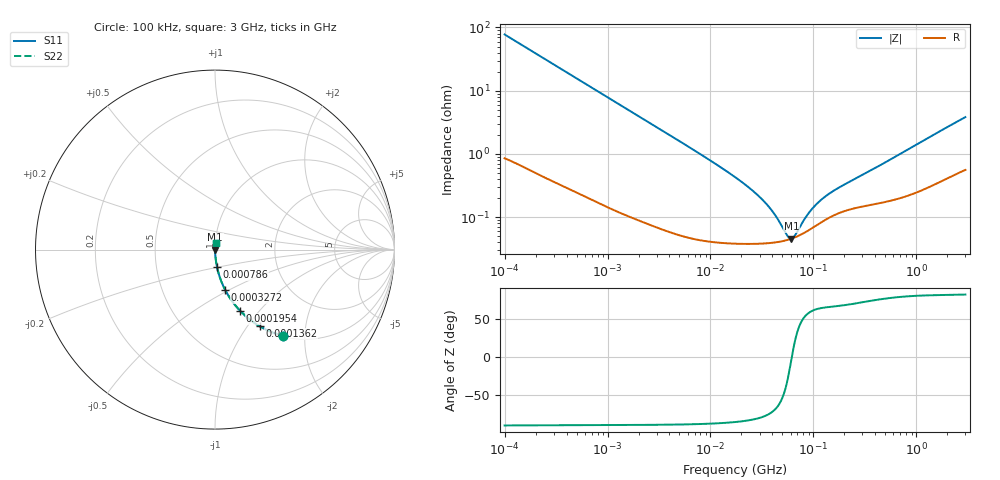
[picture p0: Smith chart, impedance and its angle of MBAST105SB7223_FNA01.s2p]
! MBAST105SB7223_FNA01  S-PARAMETER MODEL  ( Standard Model )
! Model Generated by TAIYO YUDEN Corporation (http://www.ty-top.com)
! Version 1.0
! TAIYO YUDEN Control No. 220601
! Copyright(c) 2015 TAIYO YUDEN CO.,LTD. All Rights Reserved.
! Product Description (link to TY-COMPAS)
! https://ds.yuden.co.jp/TYCOMPAS/or/detail?pn=MBAST105SB7223KFNA01&u=M
! Products Name : Multilayer Ceramic Capacitors
! Characteristics :
!  Capacitance : 0.022 [uF] , Rated Voltage : 25 [V] , TCC : X7R
!  Case Size : 1.0 x 0.5 / 0.039 x 0.02 [mm/inch] , Thickness : 0.5 / 0.02 [mm/inch]
!  (Conditions: Temperature = 25 [degC] , DC Bias Voltage = 0 [V])
! External Node Assignments :
!  1  o---| |---o  2
! GND o---------o GND
! Frequency Range : 100kHz  -  3GHz  [ 401 STEP ]
# MHZ S RI R 50
! Freq[MHz].  S11 Real  S11 Imag  S21 Real  S21 Imag  S12 Real  S12 Imag  S22 Real  S22 Imag
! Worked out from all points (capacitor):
!   401 points, 100 kHz to 3 GHz, reference 50 ohm
!   read as one part in series: C = 20.5 nF near 105.3 kHz
!   lowest |Z| = 45.8 mohm at 61.24 MHz (marker M1)
!   series resonance near 61.76 MHz, so ESL is about 320 pH
!   S11 on the Smith chart (normalised r, x): 100 kHz: 1.02, -1.55; 136.2 kHz: 1.01, -1.14; 195.4 kHz: 1.01, -0.80; 327.2 kHz: 1.01, -0.48; 786 kHz: 1.00, -0.20; 3 GHz: 1.01, +0.08
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0.1  0.3766 -0.479  0.6234 0.479  0.6234 0.479  0.3766 -0.479
0.136243  0.248 -0.4259  0.752 0.4259  0.752 0.4259  0.248 -0.4259
0.19544  0.1403 -0.341  0.8597 0.341  0.8597 0.341  0.1403 -0.341
0.327242  0.0569 -0.2247  0.9431 0.2247  0.9431 0.2247  0.0569 -0.2247
0.562235  0.0213 -0.1366  0.9787 0.1366  0.9787 0.1366  0.0213 -0.1366
0.786003  0.0116 -0.099  0.9884 0.099  0.9884 0.099  0.0116 -0.099
3.161081  0.0013 -0.0252  0.9987 0.0252  0.9987 0.0252  0.0013 -0.0252
9.331111  0.000485 -0.00843  0.9995 0.00843  0.9995 0.00843  0.000485 -0.00843
17.7727  0.000398 -0.00416  0.9996 0.00416  0.9996 0.00416  0.000398 -0.00416
25.49486  0.000385 -0.00263  0.9996 0.00263  0.9996 0.00263  0.000385 -0.00263
33.85116  0.000387 -0.00167  0.9996 0.00167  0.9996 0.00167  0.000387 -0.00167
42.68829  0.0004 -0.000992  0.9996 0.000992  0.9996 0.000992  0.0004 -0.000992
55.23785  0.000434 -0.000293  0.9996 0.000293  0.9996 0.000293  0.000434 -0.000293
58.15973  0.000445 -0.000157  0.9996 0.000157  0.9996 0.000157  0.000445 -0.000157
61.23616  0.000458 -2.19e-05  0.9995 2.19e-05  0.9995 2.19e-05  0.000458 -2.19e-05
66.15861  0.00048 0.00018  0.9995 -0.00018  0.9995 -0.00018  0.00048 0.00018
83.42988  0.000578 0.000782  0.9994 -0.000782  0.9994 -0.000782  0.000578 0.000782
97.38194  0.000674 0.00118  0.9993 -0.00118  0.9993 -0.00118  0.000674 0.00118
119.6798  0.000835 0.0017  0.9992 -0.0017  0.9992 -0.0017  0.000835 0.0017
154.8634  0.00106 0.00235  0.9989 -0.00235  0.9989 -0.00235  0.00106 0.00235
547.5153  0.00186 0.00777  0.9981 -0.00777  0.9981 -0.00777  0.00186 0.00777
3000  0.00697 0.0374  0.993 -0.0374  0.993 -0.0374  0.00697 0.0374
